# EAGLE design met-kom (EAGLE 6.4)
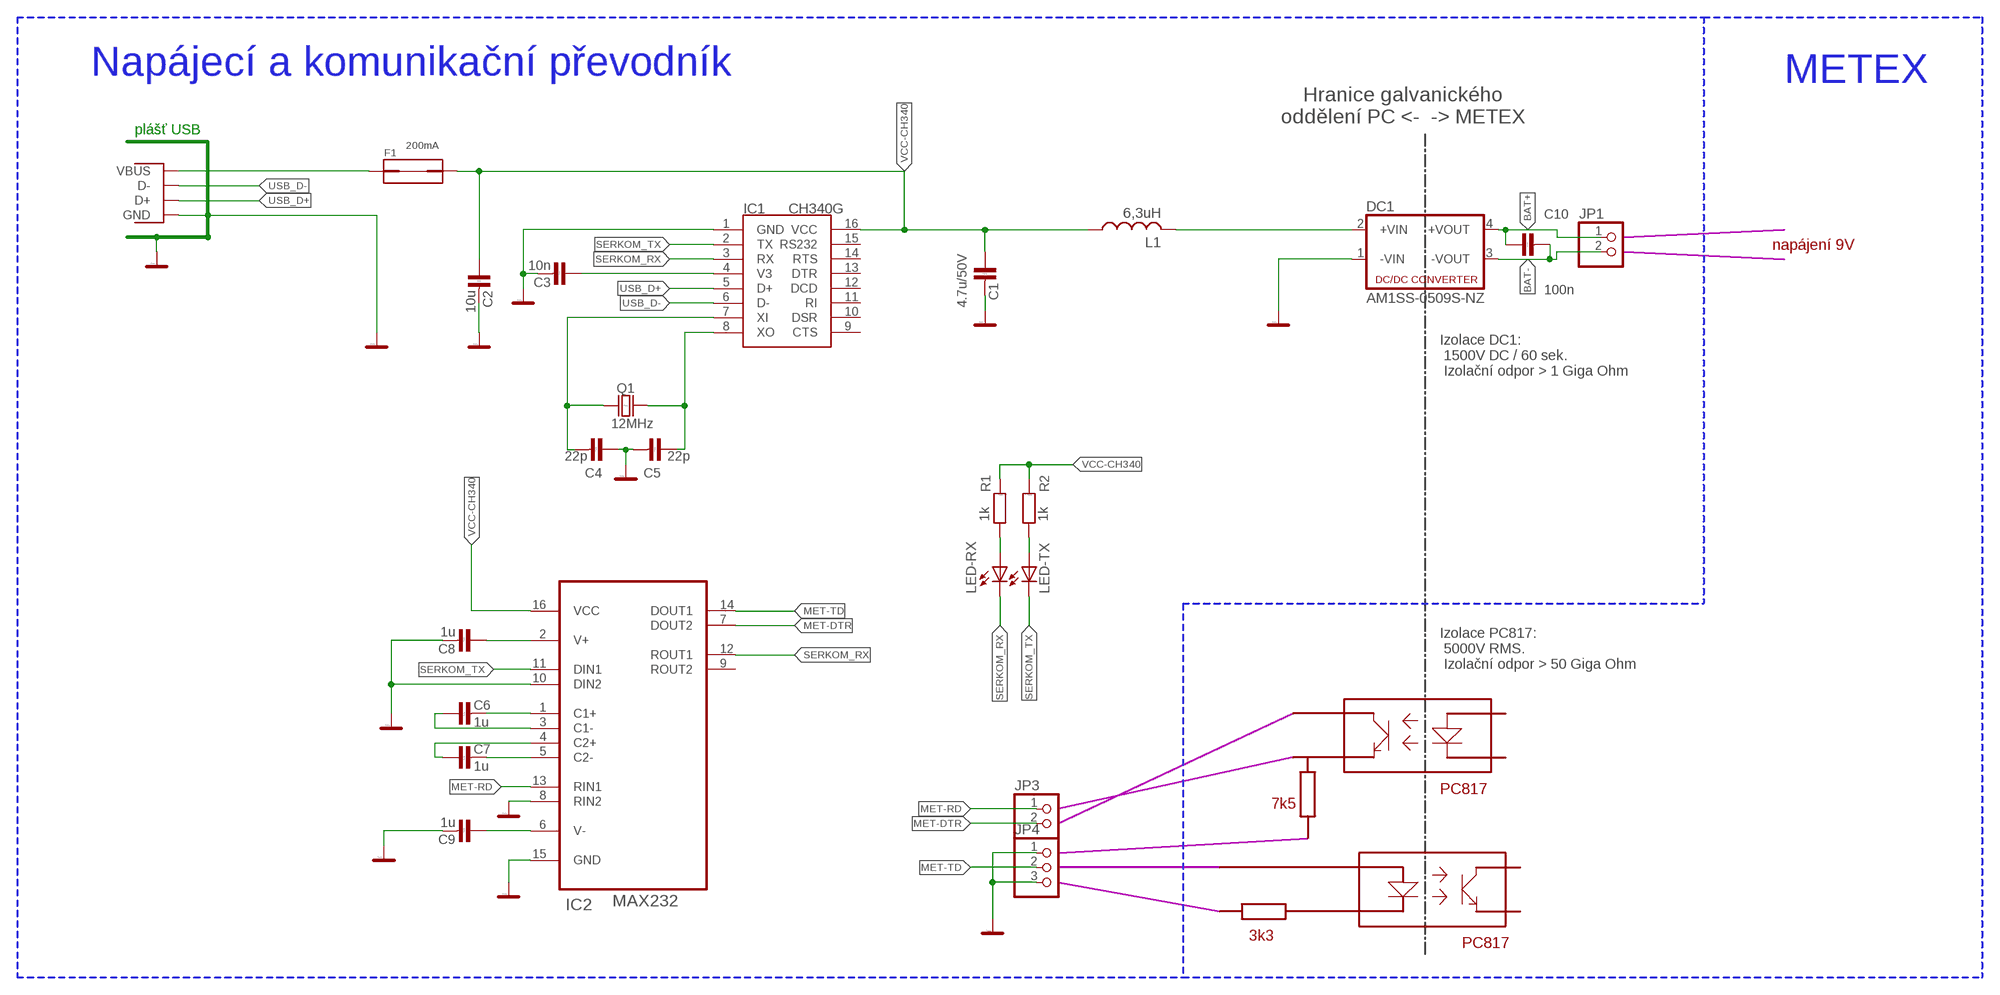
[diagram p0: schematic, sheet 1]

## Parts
C1  4.7u/50V  C-KERAMIK_SMD_0805  [0805@1]
C2  10u  C-KERAMIK_SMD_0805  [0805@1]
C3  10n  C-KERAMIK_SMD_0805  [0805@1]
C4  22p  C-KERAMIK_SMD_0805  [0805@1]
C5  22p  C-KERAMIK_SMD_0805  [0805@1]
C6  1u  C-KERAMIK_SMD_0805  [0805@1]
C7  1u  C-KERAMIK_SMD_0805  [0805@1]
C8  1u  C-KERAMIK_SMD_0805  [0805@1]
C9  1u  C-KERAMIK_SMD_0805  [0805@1]
C10  100n  C-KERAMIK_SMD_0805  [0805@1]
DC1  AM1SS-0509S-NZ  NME  [NME]
F1  200mA  FUSE1812  [FUSE1812]
IC1  CH340G  [SOIC16]
IC2  MAX232  MAX3232CDR  [SOIC127P600X175-16N]
JP1  PINHD-1X2  [1X02]
JP3  PINHD-1X2  [1X02]
JP4  PINHD-1X3  [1X03]
L1  6,3uH  L-USL0805  [L0805]
LED-RX  LEDCHIP-LED0805  [CHIP-LED0805]
LED-TX  LEDCHIP-LED0805  [CHIP-LED0805]
Q1  12MHz  Q_HC-49U  [HC-49U]
R1  1k  R_SMD_0805  [0805]
R2  1k  R_SMD_0805  [0805]
USB1  USBPTH  [USB-B-PTH]

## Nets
BAT+: C10.1 DC1.4(+VOUT) JP1.1
BAT-: C10.2 DC1.3(-VOUT) JP1.2
C1+232: C6.2 IC2.1(C1+)
C1-232: C6.1 IC2.3(C1-)
C2+232: C7.1 IC2.4(C2+)
C2-232: C7.2 IC2.5(C2-)
CH340-V3: C3.1 IC1.4(V3)
DCDC-IN: DC1.2(+VIN) L1.2
GND: C1.2 C2.2 C3.2 C4.1 C5.2 C8.2 C9.2 DC1.1(-VIN) IC1.1(GND) IC2.8(RIN2) IC2.10(DIN2) IC2.15(GND) JP4.1 JP4.3 USB1.GND
LEDR: LED-RX.A R1.1
LEDT: LED-TX.A R2.1
MET-DTR: IC2.7(DOUT2) JP3.2
MET-RD: IC2.13(RIN1) JP3.1
MET-TD: IC2.14(DOUT1) JP4.2
SERKOM_RX: IC1.3(RX) IC2.12(ROUT1) LED-RX.C
SERKOM_TX: IC1.2(TX) IC2.11(DIN1) LED-TX.C
USB_D+: IC1.5(D+) USB1.D+
USB_D-: IC1.6(D-) USB1.D-
V+232: C8.1 IC2.2(V+)
V-232: C9.1 IC2.6(V-)
V-USB-IN: F1.P$2 USB1.VBUS
VCC-CH340: C1.1 C2.1 F1.P$1 IC1.16(VCC) IC2.16(VCC) L1.1 R1.2 R2.2
XI: C4.2 IC1.7(XI) Q1.1
XO: C5.1 IC1.8(XO) Q1.2
Unconnected: IC1.9(CTS) IC1.10(DSR) IC1.11(RI) IC1.12(DCD) IC1.13(DTR) IC1.14(RTS) IC1.15(RS232) IC2.9(ROUT2)

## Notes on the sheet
- Napájecí a komunikační převodník | METEX
- Hranice galvanického
  oddělení PC <-  -> METEX
- plášť USB
- napájení 9V
- Izolace DC1:
   1500V DC / 60 sek.
   Izolační odpor > 1 Giga Ohm
- Izolace PC817:
   5000V RMS.
   Izolační odpor > 50 Giga Ohm
- PC817
- 7k5
- 3k3
- PC817

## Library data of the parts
C1-C10 = #PaJa_30:C-KERAMIK: Kondenzator - keramicky
DC1 = dc-dc-converter:NME: DC-DC CONVERTER
F1 = fuse1812:FUSE1812
IC1 = usb-serial:CH340G
IC2 = Texas Instruments_By_element14_Batch_1:MAX3232CDR: Multi Channel RS-232 Line Driver/Recevier; MPN: MAX3232CDR; OC_FARNELL: 1564957; OC_NEWARK: 35K4720; PACKAGE: SOIC-16; SUPPLIER: TEXAS INSTRUMENTS
JP1 JP3 = pinhead:PINHD-1X2: PIN HEADER
JP4 = pinhead:PINHD-1X3: PIN HEADER
L1 = rcl:L-US: INDUCTOR, American symbol
LED-RX LED-TX = led:LED: LED
Q1 = #PaJa_30:Q_HC-49U: Krystal - 1MHz - 48MHz
R1 R2 = #PaJa_30:R: Rezistor
USB1 = USB-Bx:USB: USB Connectors USB-B-PTH is fully proven SKU : PRT-00139 USB-miniB is fully proven SKU : PRT-00587 USB-A-PCB is untested. USB-A-H is C@H proven USB-B-SMT is throughly reviewed, but untested. Needs silkscreen touching up. USB-A-S has not been used/tested USB-MB-H has not been used/tested

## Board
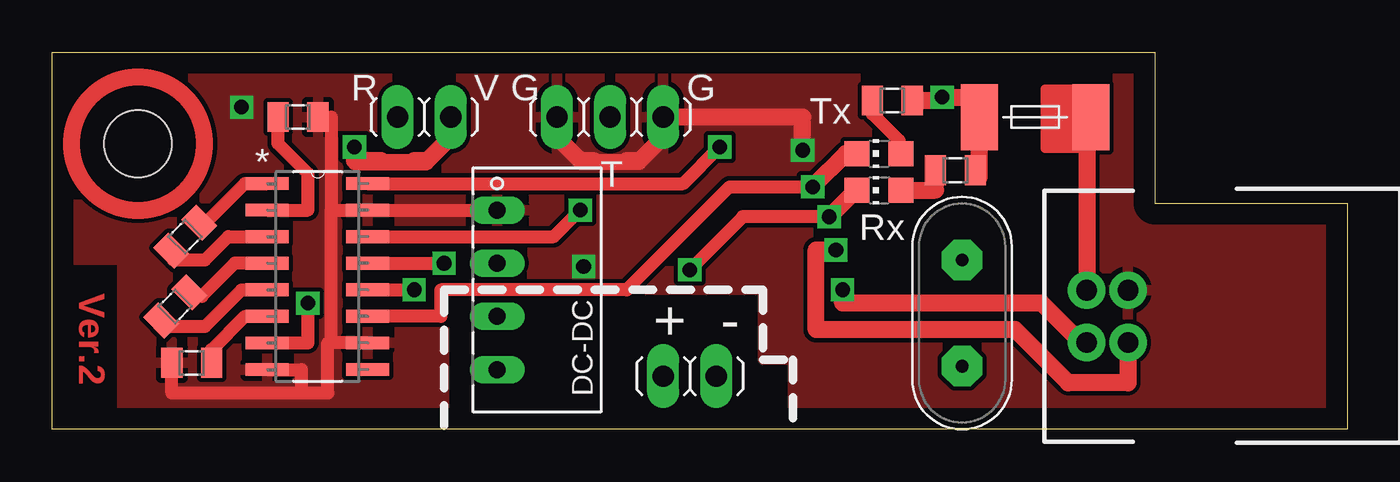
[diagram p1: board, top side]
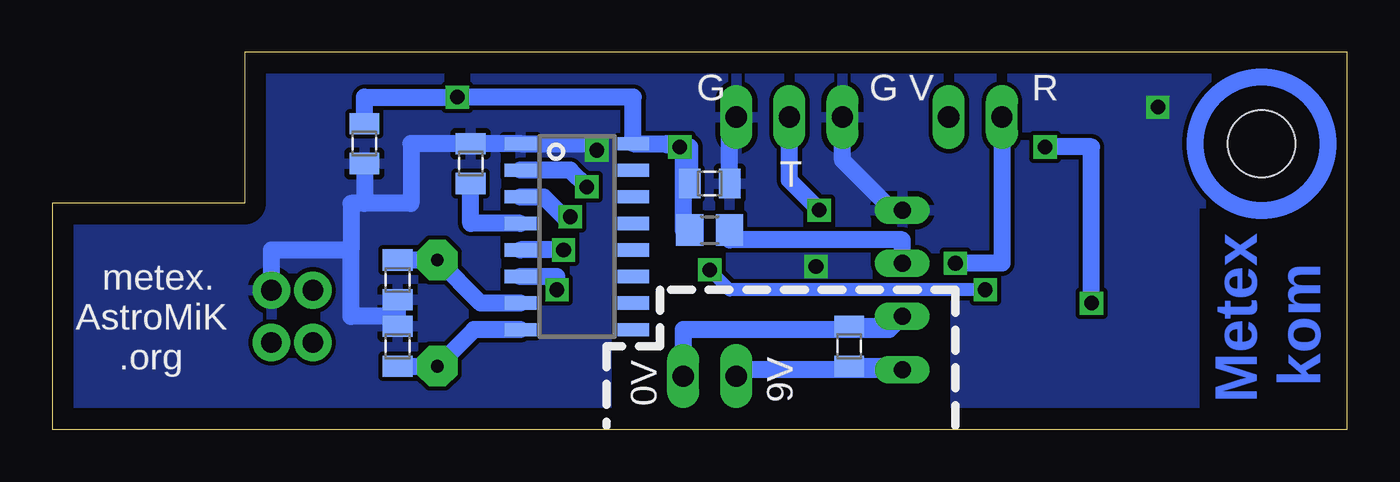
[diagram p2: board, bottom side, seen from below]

Size 61.91 x 18.02 mm. Coordinates in mm from the lower left corner, seen from the top.
Outline: 0,0 0,18.02 52.7,18.02 52.7,10.79 61.91,10.79 61.91,0 0,0
Copper layers (1*16): Top 0.035mm / dielectric 1.5mm / Bottom 0.035mm
Design rules "default *": minimum track width 10mil, minimum drill 24mil, track to track 8mil, track to pad 8mil, pad to pad 8mil, via to via 8mil, smd to smd 8mil, copper to edge 40mil, drill to drill 8mil, minimum pad ring 10mil, minimum via ring 8mil, stop-mask expansion 4mil, vias tented up to drill 0mil, thermal gap 10mil
Holes 3.2 mm at 4.1,13.65

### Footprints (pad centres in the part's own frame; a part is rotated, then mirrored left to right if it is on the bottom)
0805@1 = smd 1.016 x 1.422: 1 -0.953,0; 2 0.953,0
NME = drill 0.813 long: 1 0,3.81; 2 0,1.27; 3 0,-1.27; 4 0,-3.81
FUSE1812 = smd 1.778 x 3.15: P$1 -2.667,0; P$2 2.667,0
SOIC16 = smd 0.635 x 1.524: 1 -4.445,-2.695; 2 -3.175,-2.695; 3 -1.905,-2.695; 4 -0.635,-2.695; 5 0.635,-2.695; 6 1.905,-2.695; 7 3.175,-2.695; 8 4.445,-2.695; 9 4.445,2.695; 10 3.175,2.695; 11 1.905,2.695; 12 0.635,2.695; 13 -0.635,2.695; 14 -1.905,2.695; 15 -3.175,2.695; 16 -4.445,2.695
SOIC127P600X175-16N = smd 2.057 x 0.61: 1 -4.801,8.89; 2 -4.801,7.62; 3 -4.801,6.35; 4 -4.801,5.08; 5 -4.801,3.81; 6 -4.801,2.54; 7 -4.801,1.27; 8 -4.801,0; 9 0,0; 10 0,1.27; 11 0,2.54; 12 0,3.81; 13 0,5.08; 14 0,6.35; 15 0,7.62; 16 0,8.89
1X02 = drill 1.016 long: 1 -1.27,0; 2 1.27,0
1X03 = drill 1.016 long: 1 -2.54,0; 2 0,0; 3 2.54,0
L0805 = smd 1.3 x 1.5: 1 -0.95,0; 2 0.95,0
CHIP-LED0805 = smd 1.2 x 1.2: A 0,-1.05; C 0,1.05
HC-49U = drill 0.61 pad 1.93 octagon: 1 -2.54,0; 2 2.54,0
0805 = smd 1.016 x 1.422: 1 -0.953,0; 2 0.953,0
USB-B-PTH = drill 1 pad 1.778: D+ 0,1.25; D- 1.981,1.25; GND 0,-1.25; VBUS 1.981,-1.25

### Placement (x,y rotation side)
C1  30.48,11.75 0 bottom
C2  46.99,13.65 270 bottom
C3  41.91,12.7 90 bottom
C4  45.4,7.14 90 bottom
C5  45.4,3.97 90 bottom
C6  6.35,9.21 45 top
C7  5.87,5.87 225 top
C8  11.75,14.92 0 top
C9  6.67,3.17 180 top
C10  23.81,3.97 90 bottom
DC1  21.27,6.67 0 top
F1  46.99,14.92 0 top
IC1  36.83,9.21 270 bottom
IC2  15.08,2.86 0 top
JP1  30.48,2.54 0 top
JP3  17.78,14.92 0 top
JP4  26.67,14.92 0 top
L1  30.48,9.53 0 bottom
LED-RX  39.53,11.43 90 top
LED-TX  39.53,13.18 90 top
Q1  43.5,5.56 270 top
R1  43.18,12.38 0 top
R2  40.16,15.72 0 top
USB1  51.44,5.4 180 top

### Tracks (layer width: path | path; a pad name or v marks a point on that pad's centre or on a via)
BAT+
  Bottom 0.813: JP1.1 29.21,2.86 DC1.4 21.43,3.02 C10.1
BAT-
  Bottom 0.813: JP1.2 31.75,4.76 21.91,4.76 DC1.3 21.75,4.92 C10.2
C1+232
  Top 0.61: C6.2 7.18,9.72 9.21,11.75 IC2.1
C1-232
  Top 0.61: IC2.3 8.41,9.21 7.3,8.1 5.8,8.1 5.8,8.41 C6.1
C2+232
  Top 0.61: IC2.4 8.73,7.94 7.14,6.35 6.75,6.35 C7.1
C2-232
  Top 0.61: IC2.5 9.05,6.67 7.3,4.92 5.32,4.92 5.32,5.08 C7.2
CH340-V3
  Bottom 0.813: IC1.4 41.91,9.84 C3.1
DCDC-IN
  Bottom 0.813: DC1.2 21.27,9.05 29.53,9.05 L1.2
GND  (via drill 0.7)
  Top 0.406: C8.2 13.34,14.92
  Top 0.61: 25.88,12.86 27.46,12.86 | DC1.1 IC2.15 13.34,10.48 | 13.34,14.92 13.34,10.48 | IC2.10 13.34,4.13 | 13.34,4.13 13.34,10.48 | 11.91,1.75 5.71,1.75 C9.2 | 11.91,1.75 13.18,1.75 13.18,4.13 13.34,4.13 | 25.24,12.7 28.1,12.7 28.1,12.86 | IC2.8 11.91,2.86 11.91,1.75
  Top 0.813: v35.88,13.34 35.88,14.92 JP4.3 29.21,13.97 28.1,12.86 27.46,12.86 | JP4.1 24.13,13.97 25.24,12.86 25.88,12.86
  Bottom 0.813: C5.2 45.4,5.4 | 45.4,5.4 C4.1 | USB1.GND 51.44,8.57 47.62,8.57 | IC1.1 44.77,13.65 44.77,10.79 46.99,10.79 | 46.99,10.79 47.62,10.79 47.62,8.57 | IC1.1 C3.2 | C2.2 46.99,10.79 | IC1.1 35.88,13.65 v35.88,13.34 | 45.4,5.4 47.62,5.4 47.62,8.57 | DC1.1 21.75,10.48 24.13,12.86 JP4.1 | C1.2 29.53,14.92 JP4.3
  other vias: 9.05,15.4 25.4,7.78
  pour Bottom: 61.91,0 35.4,0 35.4,6.67 18.73,6.67 18.73,0 7.3,0 7.3,10.79 0,10.79 0,18.02 52.7,18.02 52.7,10.79 61.91,10.79
  pour Top: 61.91,0 35.4,0 35.4,3.33 33.97,3.33 33.97,6.67 18.73,6.67 18.73,0 3.33,0 3.33,8.1 0,8.1 0,18.02 52.7,18.02 52.7,10.79 61.91,10.79
LEDR
  Top 0.813: LED-RX.A 42.23,11.43 R1.1
LEDT
  Top 0.61: R2.1 39.21,15.08 40.48,13.81 40.48,13.27 LED-TX.A
MET-DTR  (via drill 0.7)
  Top 0.61: IC2.7 12.22,4.13 v12.22,6.03 | 15.72,12.86 17.3,12.86 | 19.05,13.97 JP3.2 | 14.45,12.7 17.94,12.7 17.94,12.86
  Top 0.813: 15.72,12.86 14.45,12.86 v14.45,13.49 | 17.3,12.86 17.94,12.86 19.05,13.97
  Bottom 0.813: v12.22,6.03 12.22,13.49 v14.45,13.49
MET-RD  (via drill 0.7)
  Top 0.61: IC2.13 v18.73,7.94
  Bottom 0.813: JP3.1 16.51,7.94 v18.73,7.94
MET-TD  (via drill 0.7)
  Top 0.61: IC2.14 23.97,9.21 v25.24,10.48
  Bottom 0.813: v25.24,10.48 26.67,11.91 JP4.2
SERKOM_RX  (via drill 0.7)
  Top 0.61: v37.15,10.16 33.02,10.16 v30.48,7.62 | IC2.12 v17.3,6.67 | LED-RX.C 38.42,11.43
  Top 0.813: 38.42,11.43 v37.15,10.16
  Bottom 0.61: v17.3,6.67 29.53,6.67 v30.48,7.62
  Bottom 0.813: IC1.3 38.42,11.11 37.47,10.16 v37.15,10.16
SERKOM_TX  (via drill 0.7)
  Top 0.61: v36.35,11.59 32.38,11.59 27.46,6.67 18.57,6.67 18.57,5.4 IC2.11 | LED-TX.C 37.94,13.18
  Top 0.813: 37.94,13.18 v36.35,11.59
  Bottom 0.813: IC1.2 37.15,12.38 v36.35,11.59
USB_D+  (via drill 0.7)
  Top 0.813: USB1.D+ 51.44,2.22 48.58,2.22 46.04,4.76 36.51,4.76 36.51,8.57 v37.47,8.57
  Bottom 0.813: v37.47,8.57 IC1.5
USB_D-  (via drill 0.7)
  Top 0.813: USB1.D- 49.19,4.15 47.31,6.03 37.78,6.03 v37.78,6.67
  Bottom 0.813: v37.78,6.67 37.78,7.3 IC1.6
V+232
  Top 0.61: IC2.2 12.22,10.48 12.22,12.22 10.79,13.65 C8.1 10.64,14.92
V-232
  Top 0.61: C9.1 7.62,3.81 9.21,5.4 IC2.6
V-USB-IN
  Top 0.406: 48.97,13.65 47.78,13.65 47.78,16.03 48.66,16.03 48.66,13.89 48.1,13.89 48.1,15.88 48.34,15.88 48.34,13.97 | 48.97,13.41 47.47,13.41 47.47,16.27 49.05,16.27 | 49.13,13.41 48.97,13.41 | 48.97,13.41 48.97,13.65 | 48.97,13.65 49.66,13.65 F1.P$2
  Top 0.61: 49.45,14.61 49.66,14.61 F1.P$2
  Top 0.813: 49.45,14.61 USB1.VBUS
VCC-CH340  (via drill 0.7)
  Top 0.61: IC2.16 30.16,11.75 v31.91,13.49 | 42.39,15.72 v42.55,15.88 | R1.2 44.13,12.06 44.32,12.06
  Top 0.813: v42.55,15.88 44.32,15.88 F1.P$1 44.32,12.06 | R2.2 42.39,15.72
  Bottom 0.61: v31.91,13.49 32.54,13.49 32.54,13.65 | 34.92,15.88 36.83,15.88
  Bottom 0.813: 34.13,15.88 IC1.16 32.54,13.65 31.75,13.65 31.75,9.53 L1.1 | 34.13,15.88 | 34.13,15.88 36.83,15.88 v42.55,15.88 46.99,15.88 C2.1 | C1.1 31.43,13.49 v31.91,13.49
XI
  Bottom 0.813: C4.2 Q1.1 41.43,6.03 IC1.7
XO
  Bottom 0.813: C5.1 Q1.2 41.75,4.76 IC1.8
(copper drawn outside any net)
  shapes: Bottom circle x1, Top circle x1

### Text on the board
Top: Ver.2
Bottom: Metex / kom
tPlace: R | V | G | G | Tx | T | Rx | + | -
bPlace: R | V | G | G | T | metex. | AstroMiK | .org | 9V | 0V
tStop: Ver.2
bStop: Metex / kom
